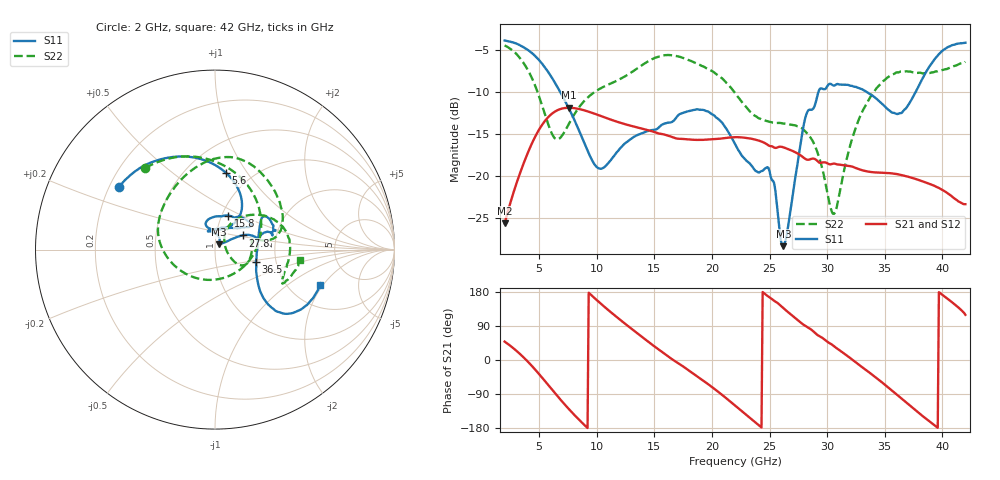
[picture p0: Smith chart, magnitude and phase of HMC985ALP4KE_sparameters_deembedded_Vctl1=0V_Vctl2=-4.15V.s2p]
!s2p File: Measurements: S11, S21, S12, S22
# GHz S dB R 50.0
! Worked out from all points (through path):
!   401 points, 2 GHz to 42 GHz, reference 50 ohm
!   highest |S21| = -11.90 dB at 7.6 GHz (marker M1); lowest = -25.7 dB at 2 GHz (marker M2)
!   lowest |S11| = -28.4 dB at 26.2 GHz (marker M3), VSWR 1.08, Z = 52.3 + j3.17 ohm
!   |S11| at or under -10 dB: 6.821 GHz to 29.25 GHz (22.43 GHz wide, 124 % of centre); 33.42 GHz to 37.69 GHz (4.271 GHz wide, 12 % of centre)
!   |S22| runs from -24.5 to -4.5 dB; largest |S21 - S12| = 0.00024
!   S11 on the Smith chart (normalised r, x): 2 GHz: 0.24, +0.28; 5.6 GHz: 0.76, +0.80; 15.8 GHz: 1.07, +0.42; 27.8 GHz: 1.34, +0.22; 36.5 GHz: 1.57, -0.23; 42 GHz: 2.94, -1.89
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2  -3.88 147.0  -25.67 48.6  -25.68 48.6  -4.47 130.5
3.6  -4.66 120.3  -18.70 8.3  -18.70 8.3  -6.48 84.9
4.7  -5.80 99.5  -15.21 -26.9  -15.22 -26.9  -9.44 43.4
5.6  -7.28 81.9  -13.29 -59.2  -13.30 -59.2  -13.09 -3.8
6.5  -9.22 66.5  -12.25 -92.1  -12.25 -92.1  -15.64 -69.3
7.6  -12.03 54.8  -11.90 -130.2  -11.90 -130.2  -13.76 -136.1
8.7  -15.38 55.0  -12.12 -164.8  -12.12 -164.9  -11.42 -170.4
10.4  -19.15 89.6  -12.90 147.3  -12.90 147.3  -9.54 162.2
15.4  -14.22 75.7  -14.96 27.2  -14.97 27.2  -5.79 86.7
15.8  -13.83 68.7  -15.06 18.3  -15.07 18.3  -5.66 81.7
19.4  -12.24 33.3  -15.70 -57.7  -15.71 -57.7  -7.09 34.6
22  -16.19 51.2  -15.40 -120.0  -15.41 -120.0  -10.13 10.0
24.9  -19.04 104.7  -16.37 167.3  -16.37 167.3  -13.53 13.2
26.2  -28.37 52.5  -16.60 136.9  -16.61 136.9  -13.77 -2.9
27.8  -15.23 27.2  -17.66 96.4  -17.66 96.4  -14.33 -25.1
28.7  -12.11 12.6  -17.95 78.3  -17.96 78.2  -15.74 -31.9
30.6  -9.26 19.5  -18.54 36.3  -18.54 36.3  -24.52 18.6
32.8  -9.59 33.9  -19.22 -13.6  -19.23 -13.6  -13.12 52.8
35.4  -12.21 11.7  -19.68 -74.9  -19.68 -74.9  -8.16 20.8
36.5  -12.47 -16.7  -19.92 -102.8  -19.92 -102.8  -7.57 6.8
39.5  -5.85 -43.7  -21.32 -176.5  -21.31 -176.5  -7.56 -26.3
42  -4.16 -18.6  -23.37 119.2  -23.39 119.2  -6.43 -6.9
